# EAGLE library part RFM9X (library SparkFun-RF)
RFM95/96/97/98 The RFM95/96/97/98(W) transceivers feature the LoRaTM long range modem that provides ultra-long range spread spectrum communication and high interference immunity whilst minimising current consumption. These devices also support high performance (G)FSK modes for systems including WMBus, IEEE802.15.4g. The RFM95/96/97/98(W) deliver exceptional phase noise, selectivity, receiver linearity and IIP3 for significantly lower current consumption than competing devices Datasheet
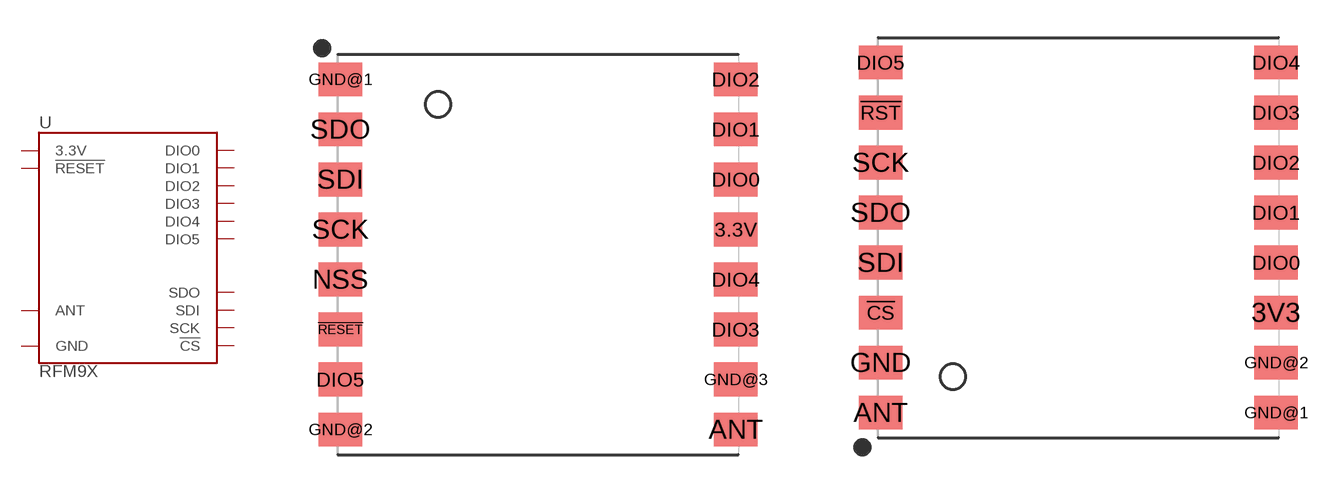
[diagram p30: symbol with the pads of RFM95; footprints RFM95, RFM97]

Designator prefix U

## RFM9XRFM95 (PROD_ID: IC-13959)  [RFM95]
3.3V  3.3V
!RESET  !RESET
ANT  ANT
DIO0  DIO0
DIO1  DIO1
DIO2  DIO2
DIO3  DIO3
DIO4  DIO4
DIO5  DIO5
GND@1  GND
GND@2  GND
GND@3  GND
NSS  !CS!
SCK  SCK
SDI  SDI
SDO  SDO

## RFM9XRFM97 (PROD_ID: IC-15944)  [RFM97]
3V3  3.3V
!CS!  !CS!
!RST  !RESET
ANT  ANT
DIO0  DIO0
DIO1  DIO1
DIO2  DIO2
DIO3  DIO3
DIO4  DIO4
DIO5  DIO5
GND  GND
GND@1  GND
GND@2  GND
SCK  SCK
SDI  SDI
SDO  SDO

## Footprint RFM95 (pad centres in mm)
RFM95/96/97/98 The RFM95/96/97/98(W) transceivers feature the LoRaTM long range modem that provides ultra-long range spread spectrum communication and high interference immunity whilst minimising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
smd 1.75 x 1.35: 3.3V 7.9,1; !RESET -7.9,-3; ANT 7.9,-7; DIO0 7.9,3; DIO1 7.9,5; DIO2 7.9,7; DIO3 7.9,-3; DIO4 7.9,-1; DIO5 -7.9,-5; GND@1 -7.9,7; GND@2 -7.9,-7; GND@3 7.9,-5; NSS -7.9,-1; SCK -7.9,1; SDI -7.9,3; SDO -7.9,5

## Footprint RFM97 (pad centres in mm)
smd 1.75 x 1.35: 3V3 7.9,-3; !CS! -7.9,-3; !RST -7.9,5; ANT -7.9,-7; DIO0 7.9,-1; DIO1 7.9,1; DIO2 7.9,3; DIO3 7.9,5; DIO4 7.9,7; DIO5 -7.9,7; GND -7.9,-5; GND@1 7.9,-7; GND@2 7.9,-5; SCK -7.9,3; SDI -7.9,-1; SDO -7.9,1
